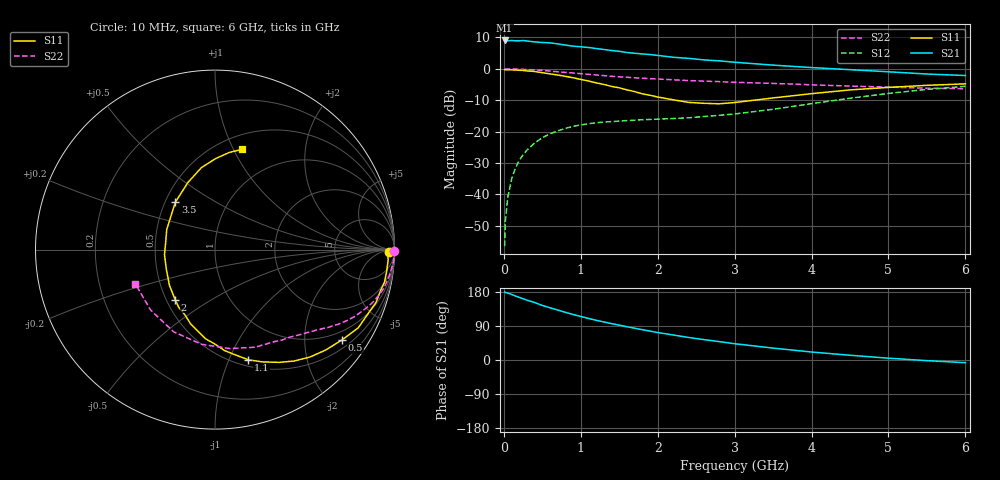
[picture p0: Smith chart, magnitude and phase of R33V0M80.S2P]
! SIEMENS Small Signal Semiconductors
! BFR181
! Si NPN RF Bipolar Junction Transistor in SOT23
! VCE = 3 V  IC = 0.8 mA
! Common Emitter S-Parameters:  May  1996
# GHz  S  MA  R  50
!  f  S11  S21  S12  S22
! GHz  MAG  ANG  MAG  ANG  MAG  ANG  MAG  ANG
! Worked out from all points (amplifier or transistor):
!   36 points, 10 MHz to 6 GHz, reference 50 ohm
!   highest |S21| = 9.1 dB at 10 MHz (marker M1)
!   |S21| within 3 dB of that: start of sweep to 1.339 GHz
!   unconditionally stable (mu >= 1): 2.128 GHz to 3.754 GHz
!   at 250 MHz: K = 0.14, MSG = 18.2 dB, |S12| = -27.4 dB
!   at 1.4 GHz: K = 0.71, MSG = 11.3 dB, |S12| = -16.8 dB
!   at 6 GHz: K = 0.88, MSG = 1.7 dB, |S12| = -5.6 dB
!   S11 on the Smith chart (normalised r, x): 10 MHz: 56, -22; 500 MHz: 0.73, -2.98; 1.1 GHz: 0.57, -1.18; 2 GHz: 0.56, -0.36; 3.5 GHz: 0.56, +0.34; 6 GHz: 0.64, +1.08
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0.01  0.9698 -0.7  2.837 179.6  0.0015 96.1  0.9983 -0.3
0.02  0.9637 -1.3  2.807 178.4  0.0038 94.2  0.9907 -0.7
0.05  0.9663 -3.5  2.801 176.6  0.0088 88.9  0.9979 -1.7
0.1  0.9642 -7.2  2.832 173.2  0.0175 84.5  0.9977 -3.3
0.15  0.9615 -10.8  2.797 168.8  0.0262 81.6  0.9927 -5.2
0.25  0.944 -18.3  2.831 161.7  0.0427 77.8  0.9832 -8.4
0.3  0.9287 -21.6  2.784 157.9  0.0509 75.4  0.976 -10.1
0.5  0.8689 -35.3  2.633 144.0  0.0801 67.0  0.9438 -16.1
0.6  0.8324 -42.3  2.596 137.9  0.0926 63.1  0.9234 -18.9
0.7  0.7991 -48.5  2.507 131.9  0.1031 59.7  0.9002 -21.5
0.9  0.7225 -60.4  2.304 120.1  0.1217 53.2  0.8606 -25.8
1.1  0.6419 -73.1  2.193 109.8  0.134 48.4  0.8189 -29.7
1.4  0.5261 -90.1  1.961 96.0  0.1446 43.4  0.7633 -34.7
1.6  0.4633 -102.1  1.823 87.7  0.1501 41.6  0.7352 -37.1
2  0.3562 -128.5  1.639 72.5  0.1585 40.7  0.6897 -42.2
2.2  0.3222 -142.0  1.532 66.1  0.1619 41.3  0.6709 -44.9
2.4  0.2927 -157.8  1.473 59.5  0.1664 43.0  0.6521 -47.6
2.8  0.278 170.6  1.342 48.5  0.1819 46.1  0.6264 -53.7
3.5  0.3444 129.9  1.148 31.4  0.2272 50.5  0.5878 -67.7
4.5  0.4625 99.5  0.972 12.5  0.3408 48.0  0.5329 -98.1
5.5  0.5472 81.6  0.828 -1.7  0.4709 35.4  0.4921 -136.8
6  0.5775 75.1  0.784 -7.1  0.5276 27.3  0.4837 -157.0
